| IBIS file 176lqfp.ibs generated by Viper version: 2014.09.14
[IBIS Ver]   4.2
[Comment Char]   |_char
[File Name]   176lqfp.ibs
[File Rev]   1
[Date]   Mon Oct  5 15:08:23 2015
[Source]   FSL Viper 2014.09.14
[Notes]
[Disclaimer] IMPORTANT NOTICE
  This information is provided on an AS IS basis and without warranty.
  IN NO EVENT SHALL Freescale BE LIABLE FOR INCIDENTAL OR CONSEQUENTIAL
  DAMAGES ARISING FROM USE OF THIS INFORMATION. THIS DISCLAIMER OF
  WARRANTY EXTENDS TO THE USER OF THE INFORMATION, AND TO THEIR CUSTOMERS
  OR USERS OF PRODUCTS  AND IS IN LIEU OF ALL WARRANTIES WHETHER EXPRESS,
  IMPLIED, OR STATUTORY, INCLUDING IMPLIED WARRANTIES OF MERCHANTABILITY
  OR FITNESS FOR PARTICULAR PURPOSE.
  Freescale does not represent or warrant that the information furnished
  hereunder is free of infringement of any third party patents,
  copyrights, trade secrets, or other intellectual property rights.
  Freescale does not represent or warrant that the information is free of
  defect, or that it meets any particular standard, requirements or need
  of the user of the infomation or their customers.
  Freescale reserves the right to change the information in this file
  without notice.
   http://www.freescale.com
[Copyright]   (C) Copyright Freescale 2004 - 2015, All Rights Reserved.
|   QFP176
[Component]   QFP176
[Manufacturer]   FREESCALE
[Package]
| variable   typ   min   max
R_pkg   0.2040288   0.0567315   0.255673
L_pkg   9.54181nH   3.84895nH   10.9689nH
C_pkg   0.40733pF   0.33943pF   1.31222pF
[Pin] signal_name   model_name   R_pin   L_pin   C_pin
1   PB_3   pad_sr_hv   0.208802  10.2363nH 0.43409pF
2   PC_9   pad_sr_hv   0.204889  10.0575nH 0.43411pF
3   PC_14   pad_sr_hv   0.201079  9.84629nH 0.43010pF
4   PC_15   pad_sr_hv   0.198237  9.59138nH 0.41496pF
5   PJ_4   pad_sr_hv   0.211864  9.57797nH 0.41218pF
6   VDD_HV_A   POWER   0.103024  7.63877nH 1.08432pF
7   VSS_HV   GND   NA   NA   NA
8   PH_15   pad_sr_hv   0.226302  9.64234nH 0.39680pF
9   PH_13   pad_sr_hv   0.220674  9.61169nH 0.39824pF
10   PH_14   pad_sr_hv   0.216824  9.55214nH 0.39232pF
11   PI_6   pad_sr_hv   0.213472  9.51616nH 0.3869pF
12   PI_7   pad_sr_hv   0.210651  9.45785nH 0.38068pF
13   PG_5   pad_sr_hv   0.208849  9.41597nH 0.37602pF
14   PG_4   pad_sr_hv   0.207444  9.4294nH  0.37109pF
15   PG_3   pad_sr_hv   0.207159  9.47344nH 0.36622pF
16   PG_2   pad_sr_hv   0.207285  9.49209nH 0.35840pF
17   PA_2   pad_sr_hv   0.210246  9.63295nH 0.34938pF
18   PE_0   pad_sr_hv   0.216042  9.64546nH 0.35030pF
19   PA_1   pad_sr_hv   0.221981  9.67998nH 0.34973pF
20   PE_1   pad_sr_hv   0.224067  9.89431nH 0.3463pF
21   PE_8   pad_sr_hv   0.23086   10.3281nH 0.34783pF
22   PE_9   pad_sr_hv   0.249945  10.8898nH 0.34482pF
23   PE_10   pad_sr_hv   0.231907  10.382nH  0.34718pF
24   PA_0   pad_sr_hv   0.216112  9.78949nH 0.35463pF
25   PE_11   pad_sr_hv   0.214723  9.73582nH 0.35074pF
26   VPP   POWER   0.143816  8.68252nH 0.37320pF
27   VDD_HV_FLA   POWER   0.144126  8.45015nH 0.37090pF
28   VSS_HV   GND   NA   NA   NA
29   RESET   BD3MSCTFRESUDQ_5V0_65U_LIN   0.204806  8.95718nH 0.35388pF
30   VDD_LP_DEC   POWER   0.18876   9.59659nH 0.64893pF
31   VDD_LV   POWER   0.120389  8.41371nH 0.38245pF
32   VRC_CTRL   NC   0.207056  9.37814nH 0.36092pF
33   PG_9   pad_sr_hv   0.208104  9.49172nH 0.37304pF
34   PG_8   pad_sr_hv   0.208037  9.58866nH 0.37743pF
35   PC_11   pad_sr_hv   0.209683  9.71531nH 0.38328pF
36   PC_10   pad_sr_hv   0.209889  9.73185nH 0.38485pF
37   PG_7   pad_sr_hv   0.211629  9.86697nH 0.39095pF
38   PG_6   pad_sr_hv   0.21403   9.98693nH 0.39736pF
39   PB_0   pad_sr_hv   0.215599  10.0908nH 0.40654pF
40   PB_1   pad_sr_hv   0.217692  10.1952nH 0.40574pF
41   PF_9   pad_sr_hv   0.214753  10.2054nH 0.40819pF
42   PF_8   pad_sr_hv   0.217519  10.2866nH 0.42622pF
43   PF_12   pad_sr_hv   0.2212   10.4529nH 0.43280pF
44   PC_6   pad_sr_hv   0.227092  10.6977nH 0.42895pF
45   PC_7   pad_sr_hv   0.207865  10.3647nH 0.43394pF
46   PF_10   pad_sr_hv   0.20295   10.1158nH 0.43740pF
47   PF_11   pad_sr_hv   0.197683  9.91301nH 0.42923pF
48   PA_15   pad_sr_hv   0.196936  9.79743nH 0.42271pF
49   PF_13   pad_sr_hv   0.195605  9.68351nH 0.42018pF
50   PA_14   pad_sr_hv   0.190061  9.4131nH  0.40871pF
51   PA_4   pad_sr_hv   0.192573  9.33615nH 0.39505pF
52   PA_13   pad_sr_hv   0.223351  9.54901nH 0.39293pF
53   PA_12   pad_sr_hv   0.218099  9.4237nH  0.39717pF
54   VDD_LV   POWER   0.142677  8.50124nH 0.41061pF
55   VSS_HV   GND   NA   NA   NA
56   XTAL   NC   0.217494  8.7989nH  0.37797pF
57   VSS_HV   GND   NA   NA   NA
58   EXTAL   NC   0.215292  8.82824nH 0.3641pF
59   VDD_HV_A   POWER   0.0567315 3.84895nH 1.31222pF
60   PB_9   ISATWINJUDQ_5V0_65U_LIN   0.210379  8.88262nH 0.35745pF
61   PB_8   ISATWINJUDQ_5V0_65U_LIN   0.209614  8.97054nH 0.35532pF
62   PB_10   pad_sr_hv   0.213669  9.04365nH 0.35081pF
63   PF_0   pad_sr_hv   0.210895  9.26836nH 0.35112pF
64   PF_1   pad_sr_hv   0.211882  9.66294nH 0.34845pF
65   PF_2   pad_sr_hv   0.217214  10.0051nH 0.34609pF
66   PF_3   pad_sr_hv   0.231417  10.4881nH 0.34366pF
67   PF_4   pad_sr_hv   0.244261  10.8017nH 0.34326pF
68   PF_5   pad_sr_hv   0.22414   10.2814nH 0.34551pF
69   PF_6   pad_sr_hv   0.215403  9.95793nH 0.34077pF
70   PF_7   pad_sr_hv   0.210222  9.66839nH 0.34281pF
71   PJ_3   pad_sr_hv   0.206349  9.51775nH 0.34774pF
72   PJ_2   pad_sr_hv   0.20381   9.37833nH 0.35058pF
73   PJ_1   pad_sr_hv   0.202812  9.28688nH 0.35172pF
74   PJ_0   pad_sr_hv   0.202959  9.06069nH 0.35434pF
75   PI_15   pad_sr_hv   0.206387  8.95232nH 0.35686pF
76   PI_14   pad_sr_hv   0.201848  9.00008nH 0.35999pF
77   PD_0   ISATWINJUDQ_5V0_65U_LIN   0.199308  9.04657nH 0.37077pF
78   PD_1   ISATWINJUDQ_5V0_65U_LIN   0.199279  9.13378nH 0.37636pF
79   PD_2   ISATWINJUDQ_5V0_65U_LIN   0.200047  9.22876nH 0.38127pF
80   PD_3   ISATWINJUDQ_5V0_65U_LIN   0.201567  9.31168nH 0.38640pF
81   PD_4   ISATWINJUDQ_5V0_65U_LIN   0.204138  9.4085nH  0.39174pF
82   PD_5   ISATWINJUDQ_5V0_65U_LIN   0.209807  9.57207nH 0.40003pF
83   PD_6   ISATWINJUDQ_5V0_65U_LIN   0.214234  9.62205nH 0.40643pF
84   PD_7   ISATWINJUDQ_5V0_65U_LIN   0.218619  9.58179nH 0.40730pF
85   VDD_HV_A   POWER   0.0567315 3.84895nH 1.31222pF
86   VSS_HV   GND   NA   NA   NA
87   PD_8   ISATWINJUDQ_5V0_65U_LIN   0.203853  9.62394nH 0.43471pF
88   PB_4   ISATWINJUDQ_5V0_65U_LIN   0.207948  9.97973nH 0.43239pF
89   VSS_HV_ADC0   GND   NA   NA   NA
90   VDD_HV_ADC0   POWER   0.138442  9.17423nH 0.45937pF
91   PB_5   ISATWINJUDQ_5V0_65U_LIN   0.202649  9.82964nH 0.43248pF
92   PB_6   ISATWINJUDQ_5V0_65U_LIN   0.196508  9.64487nH 0.42926pF
93   PB_7   ISATWINJUDQ_5V0_65U_LIN   0.192674  9.53001nH 0.41800pF
94   PD_9   ISATWINJUDQ_5V0_65U_LIN   0.191475  9.43007nH 0.41188pF
95   PD_10   ISATWINJUDQ_5V0_65U_LIN   0.188275  9.24282nH 0.40715pF
96   PB_11   pad_sr_hv   0.188078  9.03654nH 0.40082pF
97   VSS_HV_ADC1   GND   NA   NA   NA
98   VDD_HV_ADC1_REF   POWER   0.184686  8.98494nH 0.38908pF
99   VDD_HV_ADC1   POWER   0.182545  9.00353nH 0.38461pF
100   PD_12   pad_sr_hv   0.18111   8.98052nH 0.38164pF
101   PB_12   pad_sr_hv   0.180397  8.99538nH 0.37513pF
102   PD_13   pad_sr_hv   0.180884  9.0359nH  0.36696pF
103   PB_13   pad_sr_hv   0.182296  9.10414nH 0.36368pF
104   PD_14   pad_sr_hv   0.199932  9.30712nH 0.35999pF
105   PB_14   pad_sr_hv   0.202254  9.44651nH 0.35872pF
106   PD_15   pad_sr_hv   0.205641  9.64661nH 0.35349pF
107   PB_15   pad_sr_hv   0.20956   9.82055nH 0.34866pF
108   PI_8   pad_sr_hv   0.215337  10.0356nH 0.33943pF
109   INT_BAL_SELECT   NC   0.222092  10.0103nH 0.34405pF
110   VDD_LV   POWER   0.168846  9.72663nH 0.37096pF
111   PI_11   pad_sr_hv   0.253653  10.8641nH 0.34649pF
112   PI_12   pad_sr_hv   0.235259  10.2774nH 0.34857pF
113   PI_13   pad_sr_hv   0.221574  9.81242nH 0.35175pF
114   PA_3   pad_sr_hv   0.214216  9.70268nH 0.34974pF
115   PG_13   pad_sr_hv   0.209046  9.57574nH 0.35273pF
116   PG_12   pad_sr_hv   0.207447  9.50147nH 0.35781pF
117   PH_0   pad_sr_hv   0.207064  9.46689nH 0.36182pF
118   PH_1   pad_sr_hv   0.207986  9.48118nH 0.36669pF
119   PH_2   pad_sr_hv   0.209132  9.44656nH 0.37082pF
120   PH_3   pad_sr_hv   0.213069  9.59936nH 0.37054pF
121   PG_1   pad_sr_hv   0.216123  9.54688nH 0.37617pF
122   PG_0   pad_sr_hv   0.221355  9.48583nH 0.37819pF
123   VSS_HV   GND   NA   NA   NA
124   VDD_HV_B   POWER   0.135876  8.47154nH 0.75892pF
125   PF_15   pad_sr_hv   0.185348  9.29296nH 0.39093pF
126   PF_14   pad_sr_hv   0.185769  9.37553nH 0.40355pF
127   PE_13   pad_sr_hv   0.189402  9.57864nH 0.41348pF
128   PA_7   pad_sr_hv   0.192106  9.68316nH 0.42003pF
129   PA_8   pad_sr_hv   0.195361  9.80518nH 0.42366pF
130   PA_9   pad_sr_hv   0.19819   9.95633nH 0.43052pF
131   PA_10   pad_sr_hv   0.204647  10.4051nH 0.44144pF
132   PA_11   pad_sr_hv   0.21177   10.7513nH 0.43896pF
133   PE_12   pad_sr_hv   0.207372  10.356nH  0.42685pF
134   PG_14   pad_sr_hv   0.234938  10.9689nH 0.44325pF
135   PG_15   pad_sr_hv   0.230999  10.7852nH 0.44866pF
136   PE_14   pad_sr_hv   0.224783  10.4901nH 0.44190pF
137   PE_15   pad_sr_hv   0.221781  10.3349nH 0.43051pF
138   PG_10   pad_sr_hv   0.222879  10.3461nH 0.42153pF
139   PG_11   pad_sr_hv   0.221427  10.2084nH 0.41530pF
140   PH_11   pad_sr_hv   0.216639  9.87006nH 0.41016pF
141   PH_12   pad_sr_hv   0.217407  9.57684nH 0.40528pF
142   PI_5   pad_sr_hv   0.235586  9.86817nH 0.38530pF
143   PI_4   pad_sr_hv   0.230875  9.89097nH 0.38728pF
144   PC_3   pad_sr_hv   0.22719   9.88196nH 0.38177pF
145   PC_2   pad_sr_hv   0.223679  9.74211nH 0.37625pF
146   PA_5   pad_sr_hv   0.221747  9.69934nH 0.37094pF
147   PA_6   pad_sr_hv   0.219673  9.54803nH 0.37324pF
148   PH_10   pad_sr_hv   0.218088  9.43326nH 0.37255pF
149   PC_1   pad_sr_hv   0.219194  9.26369nH 0.36939pF
150   VSS_HV   GND   NA   NA   NA
151   VDD_HV_A   POWER   0.148762  8.96086nH 0.37439pF
152   VDD_LV   POWER   0.0996426 6.80374nH 1.02115pF
153   PORST   NC   0.223696  10.0401nH 0.34921pF
154   PC_0   pad_sr_hv   0.23925   10.6022nH 0.35046pF
155   PH_9   pad_sr_hv   0.255673  10.9489nH 0.34956pF
156   PE_2   pad_sr_hv   0.223509  10.0334nH 0.35526pF
157   PE_3   pad_sr_hv   0.216249  9.75922nH 0.35028pF
158   PC_5   pad_sr_hv   0.212301  9.40305nH 0.35154pF
159   PC_4   pad_sr_hv   0.211721  9.13585nH 0.35025pF
160   PE_4   pad_sr_hv   0.208931  9.09467nH 0.35233pF
161   PE_5   pad_sr_hv   0.205101  9.18063nH 0.35903pF
162   PH_4   pad_sr_hv   0.202005  9.17718nH 0.35950pF
163   PH_5   pad_sr_hv   0.200122  9.20127nH 0.36345pF
164   PH_6   pad_sr_hv   0.20009   9.30451nH 0.36514pF
165   PH_7   pad_sr_hv   0.197818  9.18684nH 0.36906pF
166   PH_8   pad_sr_hv   0.198849  9.25854nH 0.37580pF
167   PE_6   pad_sr_hv   0.200533  9.35517nH 0.38053pF
168   PE_7   pad_sr_hv   0.202331  9.4057nH  0.38631pF
169   PI_3   pad_sr_hv   0.204252  9.39921nH 0.39514pF
170   PI_2   pad_sr_hv   0.208129  9.49368nH 0.39888pF
171   PI_1   pad_sr_hv   0.212822  9.56216nH 0.40619pF
172   PI_0   pad_sr_hv   0.219966  9.72871nH 0.40216pF
173   PC_12   pad_sr_hv   0.200926  9.58727nH 0.41974pF
174   PC_13   pad_sr_hv   0.201666  9.80385nH 0.43013pF
175   PC_8   pad_sr_hv   0.204808  10.0441nH 0.43636pF
176   PB_2   pad_sr_hv   0.208611  10.2174nH 0.43282pF
[Pin Mapping]   pulldown_ref   pullup_ref
1   VSS_HV   VDD_HV_A
2   VSS_HV   VDD_HV_A
3   VSS_HV   VDD_HV_A
4   VSS_HV   VDD_HV_A
5   VSS_HV   VDD_HV_A
6   NC   VDD_HV_A
7   VSS_HV   NC
8   VSS_HV   VDD_HV_A
9   VSS_HV   VDD_HV_A
10   VSS_HV   VDD_HV_A
11   VSS_HV   VDD_HV_A
12   VSS_HV   VDD_HV_A
13   VSS_HV   VDD_HV_A
14   VSS_HV   VDD_HV_A
15   VSS_HV   VDD_HV_A
16   VSS_HV   VDD_HV_A
17   VSS_HV   VDD_HV_A
18   VSS_HV   VDD_HV_A
19   VSS_HV   VDD_HV_A
20   VSS_HV   VDD_HV_A
21   VSS_HV   VDD_HV_A
22   VSS_HV   VDD_HV_A
23   VSS_HV   VDD_HV_A
24   VSS_HV   VDD_HV_A
25   VSS_HV   VDD_HV_A
26   NC   VPP
27   NC   VDD_HV_FLA
28   VSS_HV   NC
29   VSS_HV   VDD_HV_A
30   NC   VDD_LP_DEC
31   NC   VDD_LV
32   NC   NC
33   VSS_HV   VDD_HV_A
34   VSS_HV   VDD_HV_A
35   VSS_HV   VDD_HV_A
36   VSS_HV   VDD_HV_A
37   VSS_HV   VDD_HV_A
38   VSS_HV   VDD_HV_A
39   VSS_HV   VDD_HV_A
40   VSS_HV   VDD_HV_A
41   VSS_HV   VDD_HV_A
42   VSS_HV   VDD_HV_A
43   VSS_HV   VDD_HV_A
44   VSS_HV   VDD_HV_A
45   VSS_HV   VDD_HV_A
46   VSS_HV   VDD_HV_A
47   VSS_HV   VDD_HV_A
48   VSS_HV   VDD_HV_A
49   VSS_HV   VDD_HV_A
50   VSS_HV   VDD_HV_A
51   VSS_HV   VDD_HV_A
52   VSS_HV   VDD_HV_A
53   VSS_HV   VDD_HV_A
54   NC   VDD_LV
55   VSS_HV   NC
56   NC   NC
57   VSS_HV   NC
58   NC   NC
59   NC   VDD_HV_A
60   VSS_HV   VDD_HV_A
61   VSS_HV   VDD_HV_A
62   VSS_HV   VDD_HV_A
63   VSS_HV   VDD_HV_A
64   VSS_HV   VDD_HV_A
65   VSS_HV   VDD_HV_A
66   VSS_HV   VDD_HV_A
67   VSS_HV   VDD_HV_A
68   VSS_HV   VDD_HV_A
69   VSS_HV   VDD_HV_A
70   VSS_HV   VDD_HV_A
71   VSS_HV   VDD_HV_A
72   VSS_HV   VDD_HV_A
73   VSS_HV   VDD_HV_A
74   VSS_HV   VDD_HV_A
75   VSS_HV   VDD_HV_A
76   VSS_HV   VDD_HV_A
77   VSS_HV   VDD_HV_A
78   VSS_HV   VDD_HV_A
79   VSS_HV   VDD_HV_A
80   VSS_HV   VDD_HV_A
81   VSS_HV   VDD_HV_A
82   VSS_HV   VDD_HV_A
83   VSS_HV   VDD_HV_A
84   VSS_HV   VDD_HV_A
85   NC   VDD_HV_A
86   VSS_HV   NC
87   VSS_HV   VDD_HV_A
88   VSS_HV   VDD_HV_A
89   VSS_HV_ADC0   NC
90   NC   VDD_HV_ADC0
91   VSS_HV   VDD_HV_A
92   VSS_HV   VDD_HV_A
93   VSS_HV   VDD_HV_A
94   VSS_HV   VDD_HV_A
95   VSS_HV   VDD_HV_A
96   VSS_HV   VDD_HV_A
97   VSS_HV_ADC1   NC
98   NC   VDD_HV_ADC1_REF
99   NC   VDD_HV_ADC1
100   VSS_HV   VDD_HV_A
101   VSS_HV   VDD_HV_A
102   VSS_HV   VDD_HV_A
103   VSS_HV   VDD_HV_B
104   VSS_HV   VDD_HV_B
105   VSS_HV   VDD_HV_B
106   VSS_HV   VDD_HV_B
107   VSS_HV   VDD_HV_B
108   VSS_HV   VDD_HV_B
109   NC   NC
110   NC   VDD_LV
111   VSS_HV   VDD_HV_B
112   VSS_HV   VDD_HV_B
113   VSS_HV   VDD_HV_B
114   VSS_HV   VDD_HV_B
115   VSS_HV   VDD_HV_B
116   VSS_HV   VDD_HV_B
117   VSS_HV   VDD_HV_B
118   VSS_HV   VDD_HV_B
119   VSS_HV   VDD_HV_B
120   VSS_HV   VDD_HV_B
121   VSS_HV   VDD_HV_B
122   VSS_HV   VDD_HV_B
123   VSS_HV   NC
124   NC   VDD_HV_B
125   VSS_HV   VDD_HV_B
126   VSS_HV   VDD_HV_B
127   VSS_HV   VDD_HV_B
128   VSS_HV   VDD_HV_B
129   VSS_HV   VDD_HV_B
130   VSS_HV   VDD_HV_B
131   VSS_HV   VDD_HV_B
132   VSS_HV   VDD_HV_B
133   VSS_HV   VDD_HV_B
134   VSS_HV   VDD_HV_A
135   VSS_HV   VDD_HV_A
136   VSS_HV   VDD_HV_A
137   VSS_HV   VDD_HV_A
138   VSS_HV   VDD_HV_A
139   VSS_HV   VDD_HV_A
140   VSS_HV   VDD_HV_A
141   VSS_HV   VDD_HV_A
142   VSS_HV   VDD_HV_A
143   VSS_HV   VDD_HV_A
144   VSS_HV   VDD_HV_A
145   VSS_HV   VDD_HV_A
146   VSS_HV   VDD_HV_A
147   VSS_HV   VDD_HV_A
148   VSS_HV   VDD_HV_A
149   VSS_HV   VDD_HV_A
150   VSS_HV   NC
151   NC   VDD_HV_A
152   NC   VDD_LV
153   NC   NC
154   VSS_HV   VDD_HV_A
155   VSS_HV   VDD_HV_A
156   VSS_HV   VDD_HV_A
157   VSS_HV   VDD_HV_A
158   VSS_HV   VDD_HV_A
159   VSS_HV   VDD_HV_A
160   VSS_HV   VDD_HV_A
161   VSS_HV   VDD_HV_A
162   VSS_HV   VDD_HV_A
163   VSS_HV   VDD_HV_A
164   VSS_HV   VDD_HV_A
165   VSS_HV   VDD_HV_A
166   VSS_HV   VDD_HV_A
167   VSS_HV   VDD_HV_A
168   VSS_HV   VDD_HV_A
169   VSS_HV   VDD_HV_A
170   VSS_HV   VDD_HV_A
171   VSS_HV   VDD_HV_A
172   VSS_HV   VDD_HV_A
173   VSS_HV   VDD_HV_A
174   VSS_HV   VDD_HV_A
175   VSS_HV   VDD_HV_A
176   VSS_HV   VDD_HV_A
|*   Model Selector   *
[Model Selector] BD3MSCTFRESUDQ_5V0_65U_LIN
BD3MSCTFRESUDQ_5V0_65U_LIN_0   ipp_ttl_lv=0 CMOS Receiver
BD3MSCTFRESUDQ_5V0_65U_LIN_1   ipp_ttl_lv=1 TTL  Receiver
[Model Selector] ISATWINJUDQ_5V0_65U_LIN
ISATWINJUDQ_5V0_65U_LIN_0   ipp_ttl_lv=0 ; Automotive mode receiver
ISATWINJUDQ_5V0_65U_LIN_1   ipp_ttl_lv=1 ; TTL receiver
[Model Selector] pad_sr_hv
sr11_5v   5V VDDE, full drive
sr11_3v   3.3V VDDE, full drive
sr10_5v   5V VDDE, half drive
sr10_3v   3.3V VDDE, half drive
srin_5v   5V VDDE, input
srin_3v   3.3V VDDE, input
| End [Component] QFP176
| Models and submodels in the file (10): BD3MSCTFRESUDQ_5V0_65U_LIN_0 (I/O_open_drain), BD3MSCTFRESUDQ_5V0_65U_LIN_1 (I/O_open_drain), ISATWINJUDQ_5V0_65U_LIN_0 (Input), ISATWINJUDQ_5V0_65U_LIN_1 (Input), sr10_3v (3-state), sr10_5v (3-state), sr11_3v (3-state), sr11_5v (3-state), srin_3v (Input), srin_5v (Input)
